| TEXAS INSTRUMENTS INCORPORATED
| Standard Linear and Logic Group
| IBIS Model of SN74CBT6845C
| Octal FET Bus Switch with Precharged Outputs and -2V Undershoot-
| Protection
| This file contains package information for the following:
|  SOIC 20-pin (DW) package as [Component] CBT6845C_DW
|  TSSOP 20-pin (PW) package as [Component] CBT6845C_PW
|  SSOP 20-pin (DB) package as [Component] CBT6845C_DB
|  SSOP 20-pin (DBQ) package as [Component] CBT6845C_DBQ
|  TVSOP 20-pin (DGV) package as [Component] CBT6845C_DGV
|  QFN 20-pin (RGY) package as [Component] CBT6845C_RGY
|  U*BGA 20-pin (GQN) package as [Component] CBT6845C_GQN
| This device can be powered at the following Vccs:
|  5 volt Vcc
|  4 volt Vcc
| This file provides unique models under the [Model Selector] for each Vcc.
| For operation at a specific Vcc, select the appropriate model after each
| [Model Selector] keyword.
[IBIS Ver]   3.2
[Comment char]  |_char
[File Name]   sn74cbt6845c.ibs
[File Rev]   1.1 | b_die
[Date]   July 8, 2003
[Source]   Data created from TI-SPICE simulations at TI-SLL.
[Notes]   The following is an IBIS list for the CBT6845C.
   Please contact sllibis@ti.com with questions and
   comments concerning SLL IBIS models.
   - Power-clamp data has been deleted since there is no
   power-clamp diode in the device.
   - Non-monotonic data due to FET characteristics.
   - GQN package is package preview only at this date.
[Disclaimer] Property of Texas Instruments Incorporated.  Unauthorized
   reproduction and/or distribution is strictly prohibited.
   This product is protected under copyright law.
   Created  2003, (C) Copyright  2003, Texas Instruments
   Incorporated, All Rights Reserved
   UNLESS THERE IS A SIGNED, WRITTEN AGREEMENT TO THE
   CONTRARY, TEXAS INSTRUMENTS (TI) IS PROVIDING THE IBIS
   MODELS  AND WITHOUT ANY WARRANTY, EXPRESSED OR
   IMPLIED.  TI assumes no liability for:
   1) the accuracy of the IBIS models provided to your
   company;
   2) the proper functioning of these IBIS Models in your
   design or for any resulting applications; or
   3) infringement of patents, copyrights or intellectual
   property rights resulting from your use of these IBIS
   models.
   TI provides IBIS Models as a service to our customers.
   You and your company shall not distribute, sell or give
   these models to anyone else without prior written
   permission from TI.
   TI reserves the right to make changes to our products or
   to discontinue any semiconductor product or service
   without notice, and advises our customers to obtain the
   latest version of relevant information to verify, before
   placing orders, that the information being relied on is
   current.
   Please be aware that your receipt and use of the IBIS
   information provided shall serve as acceptance of these
   terms and conditions.  If you do not accept these terms,
   you should return or destroy the IBIS models and any
   other accompanying information immediately.
| Component CBT6845C_DW 20-pin SOIC
[Component]   CBT6845C_DW
[Manufacturer]   Texas Instruments, Inc.
[Package]
|   typ   min   max
R_pkg   3.800e-02   3.300e-02   4.500e-02
L_pkg   5.012e-09   4.110e-09   6.349e-09
C_pkg   7.170e-13   5.300e-13   8.680e-13
[Pin]   signal_name   model_name   R_pin   L_pin   C_pin
1   biasv   POWER   4.200e-02   6.336e-09   8.650e-13
2   a1   CBT6845C_IO   4.300e-02   5.542e-09   8.670e-13
3   a2   CBT6845C_IO   3.400e-02   4.714e-09   7.320e-13
4   a3   CBT6845C_IO   3.400e-02   4.377e-09   5.910e-13
5   a4   CBT6845C_IO   3.600e-02   4.130e-09   5.330e-13
6   a5   CBT6845C_IO   3.500e-02   4.111e-09   5.300e-13
7   a6   CBT6845C_IO   3.400e-02   4.284e-09   5.830e-13
8   a7   CBT6845C_IO   3.400e-02   4.634e-09   7.260e-13
9   a8   CBT6845C_IO   4.000e-02   5.518e-09   8.650e-13
10   GND   GND   4.300e-02   6.349e-09   8.660e-13
11   b8   CBT6845C_IO   4.100e-02   6.281e-09   8.610e-13
12   b7   CBT6845C_IO   4.500e-02   5.561e-09   8.680e-13
13   b6   CBT6845C_IO   3.300e-02   4.778e-09   7.420e-13
14   b5   CBT6845C_IO   3.500e-02   4.414e-09   5.960e-13
15   b4   CBT6845C_IO   3.500e-02   4.110e-09   5.330e-13
16   b3   CBT6845C_IO   3.600e-02   4.130e-09   5.330e-13
17   b2   CBT6845C_IO   3.400e-02   4.377e-09   5.910e-13
18   b1   CBT6845C_IO   3.400e-02   4.714e-09   7.310e-13
19   noe   CBT6845C_IN   4.300e-02   5.569e-09   8.680e-13
20   VCC   POWER   4.200e-02   6.308e-09   8.640e-13
| Component CBT6845C_PW 20-pin TSSOP
[Component]   CBT6845C_PW
[Manufacturer]   Texas Instruments, Inc.
[Package]
|   typ   min   max
R_pkg   5.000e-02   4.200e-02   6.000e-02
L_pkg   2.802e-09   2.248e-09   3.553e-09
C_pkg   3.170e-13   2.020e-13   4.430e-13
[Pin]   signal_name   model_name   R_pin   L_pin   C_pin
1   biasv   POWER   5.500e-02   3.461e-09   4.400e-13
2   a1   CBT6845C_IO   5.500e-02   3.150e-09   4.010e-13
3   a2   CBT6845C_IO   4.200e-02   2.619e-09   3.020e-13
4   a3   CBT6845C_IO   4.500e-02   2.273e-09   2.020e-13
5   a4   CBT6845C_IO   4.500e-02   2.248e-09   2.240e-13
6   a5   CBT6845C_IO   4.500e-02   2.273e-09   2.260e-13
7   a6   CBT6845C_IO   4.400e-02   2.323e-09   2.050e-13
8   a7   CBT6845C_IO   4.600e-02   2.704e-09   3.070e-13
9   a8   CBT6845C_IO   6.000e-02   3.265e-09   4.110e-13
10   GND   GND   5.700e-02   3.506e-09   4.360e-13
11   b8   CBT6845C_IO   5.800e-02   3.553e-09   4.370e-13
12   b7   CBT6845C_IO   5.800e-02   3.193e-09   4.050e-13
13   b6   CBT6845C_IO   4.200e-02   2.704e-09   3.110e-13
14   b5   CBT6845C_IO   4.600e-02   2.392e-09   2.100e-13
15   b4   CBT6845C_IO   4.700e-02   2.334e-09   2.290e-13
16   b3   CBT6845C_IO   4.700e-02   2.300e-09   2.270e-13
17   b2   CBT6845C_IO   4.700e-02   2.349e-09   2.070e-13
18   b1   CBT6845C_IO   4.500e-02   2.677e-09   3.060e-13
19   noe   CBT6845C_IN   6.000e-02   3.235e-09   4.060e-13
20   VCC   POWER   5.600e-02   3.487e-09   4.430e-13
| Component CBT6845C_DB 20-pin SSOP
[Component]   CBT6845C_DB
[Manufacturer]   Texas Instruments, Inc.
[Package]
|   typ   min   max
R_pkg   4.000e-02   3.500e-02   5.100e-02
L_pkg   3.495e-09   3.035e-09   4.314e-09
C_pkg   4.200e-13   3.460e-13   5.020e-13
[Pin]   signal_name   model_name   R_pin   L_pin   C_pin
1   biasv   POWER   4.900e-02   4.310e-09   5.020e-13
2   a1   CBT6845C_IO   4.800e-02   3.903e-09   4.870e-13
3   a2   CBT6845C_IO   3.500e-02   3.189e-09   3.960e-13
4   a3   CBT6845C_IO   3.500e-02   3.036e-09   3.470e-13
5   a4   CBT6845C_IO   3.500e-02   3.035e-09   3.670e-13
6   a5   CBT6845C_IO   3.500e-02   3.035e-09   3.670e-13
7   a6   CBT6845C_IO   3.500e-02   3.036e-09   3.470e-13
8   a7   CBT6845C_IO   3.500e-02   3.189e-09   3.970e-13
9   a8   CBT6845C_IO   4.700e-02   3.899e-09   4.880e-13
10   GND   GND   5.100e-02   4.314e-09   5.000e-13
11   b8   CBT6845C_IO   5.100e-02   4.314e-09   5.000e-13
12   b7   CBT6845C_IO   4.700e-02   3.899e-09   4.880e-13
13   b6   CBT6845C_IO   3.500e-02   3.189e-09   3.970e-13
14   b5   CBT6845C_IO   3.500e-02   3.036e-09   3.460e-13
15   b4   CBT6845C_IO   3.500e-02   3.035e-09   3.670e-13
16   b3   CBT6845C_IO   3.500e-02   3.035e-09   3.670e-13
17   b2   CBT6845C_IO   3.500e-02   3.036e-09   3.460e-13
18   b1   CBT6845C_IO   3.500e-02   3.189e-09   3.970e-13
19   noe   CBT6845C_IN   4.700e-02   3.899e-09   4.880e-13
20   VCC   POWER   5.100e-02   4.314e-09   5.020e-13
| Component CBT6845C_DBQ 20-pin SSOP
[Component]   CBT6845C_DBQ
[Manufacturer]   Texas Instruments, Inc.
[Package]
|   typ   min   max
R_pkg   3.900e-02   3.100e-02   5.000e-02
L_pkg   2.804e-09   2.292e-09   3.805e-09
C_pkg   2.940e-13   2.220e-13   4.170e-13
[Pin]   signal_name   model_name   R_pin   L_pin   C_pin
1   biasv   POWER   4.800e-02   3.760e-09   4.140e-13
2   a1   CBT6845C_IO   4.800e-02   3.053e-09   3.500e-13
3   a2   CBT6845C_IO   3.500e-02   2.506e-09   2.530e-13
4   a3   CBT6845C_IO   3.300e-02   2.368e-09   2.250e-13
5   a4   CBT6845C_IO   3.200e-02   2.302e-09   2.260e-13
6   a5   CBT6845C_IO   3.200e-02   2.303e-09   2.260e-13
7   a6   CBT6845C_IO   3.300e-02   2.368e-09   2.250e-13
8   a7   CBT6845C_IO   3.500e-02   2.506e-09   2.530e-13
9   a8   CBT6845C_IO   4.800e-02   3.053e-09   3.490e-13
10   GND   GND   4.200e-02   3.572e-09   4.040e-13
11   b8   CBT6845C_IO   4.700e-02   3.731e-09   4.140e-13
12   b7   CBT6845C_IO   4.900e-02   3.095e-09   3.550e-13
13   b6   CBT6845C_IO   4.000e-02   2.616e-09   2.590e-13
14   b5   CBT6845C_IO   3.300e-02   2.336e-09   2.220e-13
15   b4   CBT6845C_IO   3.300e-02   2.292e-09   2.250e-13
16   b3   CBT6845C_IO   3.300e-02   2.313e-09   2.270e-13
17   b2   CBT6845C_IO   3.100e-02   2.350e-09   2.230e-13
18   b1   CBT6845C_IO   4.000e-02   2.630e-09   2.600e-13
19   noe   CBT6845C_IN   4.900e-02   3.109e-09   3.550e-13
20   VCC   POWER   5.000e-02   3.805e-09   4.170e-13
| Component CBT6845C_DGV 20-pin TVSOP
[Component]   CBT6845C_DGV
[Manufacturer]   Texas Instruments, Inc.
[Package]
|   typ   min   max
R_pkg   4.400e-02   3.800e-02   4.800e-02
L_pkg   2.561e-09   2.236e-09   2.961e-09
C_pkg   3.420e-13   2.640e-13   4.460e-13
[Pin]   signal_name   model_name   R_pin   L_pin   C_pin
1   biasv   POWER   4.400e-02   2.935e-09   4.170e-13
2   a1   CBT6845C_IO   4.200e-02   2.869e-09   4.460e-13
3   a2   CBT6845C_IO   4.300e-02   2.399e-09   3.160e-13
4   a3   CBT6845C_IO   4.400e-02   2.236e-09   2.650e-13
5   a4   CBT6845C_IO   4.600e-02   2.278e-09   2.640e-13
6   a5   CBT6845C_IO   4.500e-02   2.274e-09   2.640e-13
7   a6   CBT6845C_IO   4.400e-02   2.285e-09   2.690e-13
8   a7   CBT6845C_IO   4.300e-02   2.452e-09   3.200e-13
9   a8   CBT6845C_IO   4.400e-02   2.900e-09   4.460e-13
10   GND   GND   4.400e-02   2.961e-09   4.180e-13
11   b8   CBT6845C_IO   4.500e-02   2.954e-09   4.180e-13
12   b7   CBT6845C_IO   4.200e-02   2.847e-09   4.430e-13
13   b6   CBT6845C_IO   4.500e-02   2.453e-09   3.190e-13
14   b5   CBT6845C_IO   4.500e-02   2.297e-09   2.690e-13
15   b4   CBT6845C_IO   4.800e-02   2.334e-09   2.680e-13
16   b3   CBT6845C_IO   4.800e-02   2.335e-09   2.670e-13
17   b2   CBT6845C_IO   4.600e-02   2.299e-09   2.680e-13
18   b1   CBT6845C_IO   4.600e-02   2.457e-09   3.200e-13
19   noe   CBT6845C_IN   4.300e-02   2.848e-09   4.410e-13
20   VCC   POWER   3.800e-02   2.812e-09   4.080e-13
| Component CBT6845C_RGY 20-pin QFN
[Component]   CBT6845C_RGY
[Manufacturer]   Texas Instruments, Inc.
[Package]
|   typ   min   max
R_pkg   4.600e-02   3.500e-02   5.800e-02
L_pkg   1.131e-09   8.800e-10   1.396e-09
C_pkg   1.650e-13   1.420e-13   1.750e-13
[Pin]   signal_name   model_name   R_pin   L_pin   C_pin
1   biasv   POWER   5.300e-02   1.289e-09   1.420e-13
2   a1   CBT6845C_IO   5.800e-02   1.386e-09   1.720e-13
3   a2   CBT6845C_IO   4.600e-02   1.111e-09   1.730e-13
4   a3   CBT6845C_IO   3.900e-02   9.650e-10   1.610e-13
5   a4   CBT6845C_IO   3.500e-02   8.810e-10   1.650e-13
6   a5   CBT6845C_IO   3.500e-02   8.800e-10   1.650e-13
7   a6   CBT6845C_IO   3.900e-02   9.610e-10   1.610e-13
8   a7   CBT6845C_IO   4.500e-02   1.105e-09   1.720e-13
9   a8   CBT6845C_IO   5.800e-02   1.386e-09   1.720e-13
10   GND   GND   5.600e-02   1.352e-09   1.590e-13
11   b8   CBT6845C_IO   5.300e-02   1.287e-09   1.550e-13
12   b7   CBT6845C_IO   5.800e-02   1.396e-09   1.720e-13
13   b6   CBT6845C_IO   4.700e-02   1.129e-09   1.750e-13
14   b5   CBT6845C_IO   4.000e-02   9.760e-10   1.640e-13
15   b4   CBT6845C_IO   3.500e-02   8.840e-10   1.690e-13
16   b3   CBT6845C_IO   3.500e-02   8.810e-10   1.680e-13
17   b2   CBT6845C_IO   3.900e-02   9.670e-10   1.620e-13
18   b1   CBT6845C_IO   4.600e-02   1.118e-09   1.740e-13
19   noe   CBT6845C_IN   5.800e-02   1.396e-09   1.750e-13
20   VCC   POWER   5.200e-02   1.276e-09   1.440e-13
| Component CBT6845C_GQN 20-pin U*BGA
[Component]   CBT6845C_GQN
[Manufacturer]   Texas Instruments, Inc.
[Package]
|   typ   min   max
R_pkg   4.300e-02   3.300e-02   6.100e-02
L_pkg   1.317e-09   8.960e-10   2.088e-09
C_pkg   1.130e-13   6.400e-14   1.900e-13
[Pin]   signal_name   model_name   R_pin   L_pin   C_pin
1   biasv   POWER   3.800e-02   1.199e-09   1.210e-13
2   a1   CBT6845C_IO   4.000e-02   1.067e-09   1.020e-13
3   a2   CBT6845C_IO   6.100e-02   1.999e-09   1.900e-13
4   a3   CBT6845C_IO   3.300e-02   9.630e-10   7.100e-14
5   a4   CBT6845C_IO   4.900e-02   1.523e-09   1.230e-13
6   a5   CBT6845C_IO   3.300e-02   8.960e-10   6.400e-14
7   a6   CBT6845C_IO   6.100e-02   1.899e-09   1.640e-13
8   a7   CBT6845C_IO   3.300e-02   8.980e-10   6.700e-14
9   a8   CBT6845C_IO   4.900e-02   1.514e-09   1.280e-13
10   GND   GND   3.600e-02   1.006e-09   9.400e-14
11   b8   CBT6845C_IO   4.900e-02   1.683e-09   1.460e-13
12   b7   CBT6845C_IO   3.300e-02   1.121e-09   8.900e-14
13   b6   CBT6845C_IO   6.100e-02   2.088e-09   1.730e-13
14   b5   CBT6845C_IO   3.300e-02   1.027e-09   7.100e-14
15   b4   CBT6845C_IO   4.900e-02   1.558e-09   1.240e-13
16   b3   CBT6845C_IO   3.300e-02   9.280e-10   6.700e-14
17   b2   CBT6845C_IO   6.100e-02   1.921e-09   1.770e-13
18   b1   CBT6845C_IO   3.300e-02   9.010e-10   7.700e-14
19   noe   CBT6845C_IN   3.700e-02   9.900e-10   9.800e-14
20   VCC   POWER   3.500e-02   1.168e-09   1.190e-13
[Series Switch Groups]
| Function Group States
On  1 /   | a1-a8->b1-b8 noe low
Off 1 /   | noe high, precharge all
[Series Pin Mapping]   pin_2   model_name   function_table_group
2   18   CBT6845C_IO_50_S   1
| 2   18   CBT6845C_IO_40_S   1
3   17   CBT6845C_IO_50_S   1
| 3   17   CBT6845C_IO_40_S   1
4   16   CBT6845C_IO_50_S   1
| 4   16   CBT6845C_IO_40_S   1
5   15   CBT6845C_IO_50_S   1
| 5   15   CBT6845C_IO_40_S   1
6   14   CBT6845C_IO_50_S   1
| 6   14   CBT6845C_IO_40_S   1
7   13   CBT6845C_IO_50_S   1
| 7   13   CBT6845C_IO_40_S   1
8   12   CBT6845C_IO_50_S   1
| 8   12   CBT6845C_IO_40_S   1
9   11   CBT6845C_IO_50_S   1
| 9   11   CBT6845C_IO_40_S   1
| Model CBT6845C_IN
[Model Selector]   CBT6845C_IN
CBT6845C_IN_50   5 volt Vcc
CBT6845C_IN_40   4 volt Vcc
| Model CBT6845C_IO
[Model Selector]   CBT6845C_IO
CBT6845C_IO_50   5 volt Vcc
CBT6845C_IO_40   4 volt Vcc
| Model CBT6845C_IO_S
[Model Selector]   CBT6845C_IO_S
CBT6845C_IO_50_S   5 volt Vcc_S
CBT6845C_IO_40_S   4 volt Vcc_S
[Model]   CBT6845C_IO_50_S
Model_type  Series_switch
| variable   typ   min   max
C_comp   0   0   0
[Temperature Range]   40   100   -40
| Ambient temperature   25   85   -40
[Voltage range]   5   4.5   5.5
[On]
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[Off]
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[Model]   CBT6845C_IO_40_S
Model_type  Series_switch
| variable   typ   min   max
C_comp   0   0   0
[Temperature Range]   40   100   -40
| Ambient temperature   25   85   -40
[Voltage range]   4   4   4
[On]
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[Off]
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| Models and submodels in the file (6): CBT6845C_IN_50 (Input), CBT6845C_IN_40 (Input), CBT6845C_IO_50_S (Series_switch), CBT6845C_IO_50 (Terminator), CBT6845C_IO_40_S (Series_switch), CBT6845C_IO_40 (Terminator)
